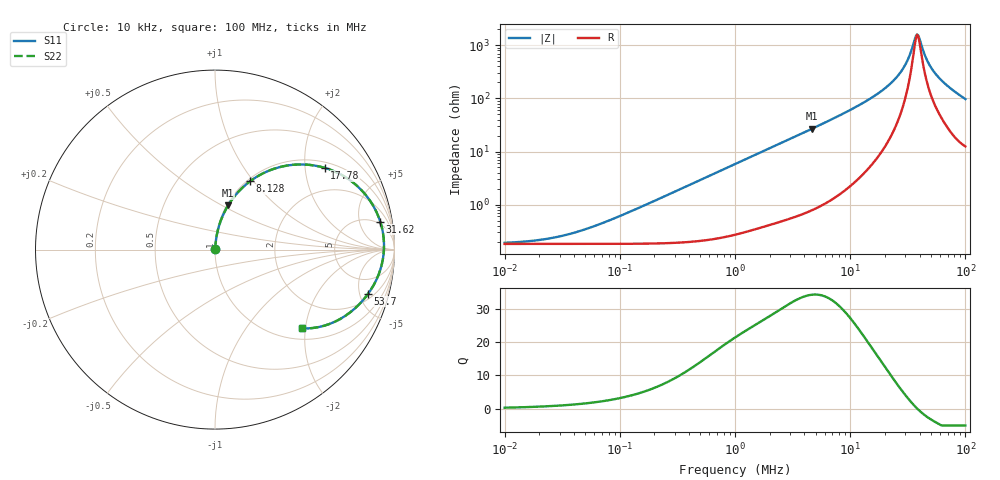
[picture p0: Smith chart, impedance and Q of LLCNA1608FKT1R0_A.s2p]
! LLCNA1608FKT1R0_A  S-PARAMETER MODEL  ( Standard Model )
! Model Generated by TAIYO YUDEN Corporation (http://www.ty-top.com)
! Version 1.0
! TAIYO YUDEN Control No. 170927
! Copyright(c) 2017 TAIYO YUDEN CO.,LTD. All Rights Reserved.
! Product Description (link to TY-COMPAS)
! https://ds.yuden.co.jp/TYCOMPAS/or/detail?pn=LLCNA1608FKT1R0MA&u=M
! Products Name : Inductors
! Characteristics :
!  Inductance : 1.0 [uH] , SRF(min) : - [Hz] , DC Resistance(max) : 224 [mOhm]
!  Rated Current : Saturation  1.5 [A] (dL = 30 [%]), Temp Rise  0.9 [A] (dT = 40 [degC])
!  Case Size : 1.6 x 0.8 / 0.063 x 0.031 [mm/inch] , Thickness : 0.6 / 0.024 [mm/inch]
!  (Conditions: Temperature = 25 [degC] , DC Bias Current = 0 [A])
! External Node Assignments :
!  1  o---GGG---o  2
! GND o---------o GND
! Frequency Range : 10kHz  -  100MHz  [ 402 STEP ]
# MHz S RI R 50
! Freq[MHz].  S11 Real  S11 Imag  S21 Real  S21 Imag  S12 Real  S12 Imag  S22 Real  S22 Imag
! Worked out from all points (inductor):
!   401 points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, 10 kHz to 100 MHz, reference 50 ohm
!   read as one part in series: L = 925 nH near 95.5 kHz
!   highest Q = 34.2 at 4.677 MHz (marker M1), where L = 915 nH
!   self-resonance near 38.32 MHz
!   S11 on the Smith chart (normalised r, x): 10 kHz: 1.00, +0.00; 8.128 MHz: 1.03, +0.96; 17.78 MHz: 1.17, +2.54; 31.62 MHz: 4, +10; 53.7 MHz: 2.58, -6.01; 100 MHz: 1.25, -1.93
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0.01  0.00182 0.000578  0.9982 -0.000578  0.9982 -0.000578  0.00182 0.000578
0.022909  0.00182 0.00132  0.9982 -0.00132  0.9982 -0.00132  0.00182 0.00132
0.046774  0.00182 0.00271  0.9982 -0.00271  0.9982 -0.00271  0.00182 0.00271
0.087096  0.00185 0.00504  0.9982 -0.00504  0.9982 -0.00504  0.00185 0.00504
0.218776  0.00202 0.0127  0.998 -0.0127  0.998 -0.0127  0.00202 0.0127
1  0.006 0.0573  0.994 -0.0573  0.994 -0.0573  0.006 0.0573
2.290868  0.0212 0.1278  0.9788 -0.1278  0.9788 -0.1278  0.0212 0.1278
4.677351  0.0737 0.2471  0.9263 -0.2471  0.9263 -0.2471  0.0737 0.2471
8.128305  0.1954 0.3805  0.8046 -0.3805  0.8046 -0.3805  0.1954 0.3805
12.8825  0.4053 0.4689  0.5947 -0.4689  0.5947 -0.4689  0.4053 0.4689
17.78279  0.6117 0.4554  0.3883 -0.4554  0.3883 -0.4554  0.6117 0.4554
21.87762  0.7484 0.3894  0.2516 -0.3894  0.2516 -0.3894  0.7484 0.3894
26.91535  0.8627 0.2738  0.1373 -0.2738  0.1373 -0.2738  0.8627 0.2738
31.62278  0.9206 0.1558  0.0794 -0.1558  0.0794 -0.1558  0.9206 0.1558
36.30781  0.941 0.044  0.059 -0.044  0.059 -0.044  0.941 0.044
38.01894  0.9414 0.00618  0.0586 -0.00618  0.0586 -0.00618  0.9414 0.00618
38.90451  0.9403 -0.0126  0.0597 0.0126  0.0597 0.0126  0.9403 -0.0126
39.81072  0.9385 -0.0312  0.0615 0.0312  0.0615 0.0312  0.9385 -0.0312
45.70882  0.912 -0.138  0.088 0.138  0.088 0.138  0.912 -0.138
53.70318  0.8536 -0.2455  0.1464 0.2455  0.1464 0.2455  0.8536 -0.2455
70.79458  0.7094 -0.3797  0.2906 0.3797  0.2906 0.3797  0.7094 -0.3797
100  0.4873 -0.4394  0.5127 0.4394  0.5127 0.4394  0.4873 -0.4394
